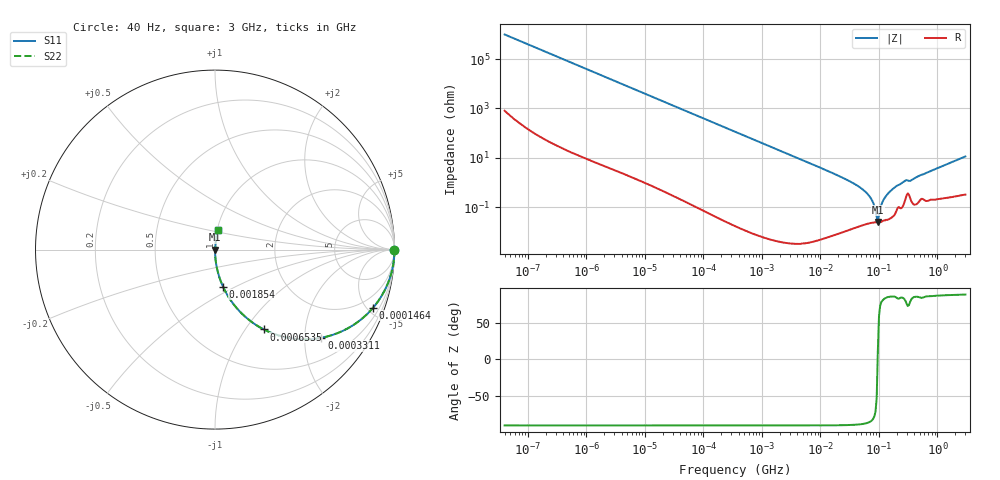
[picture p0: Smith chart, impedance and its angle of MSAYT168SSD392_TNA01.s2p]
! MSAYT168SSD392_TNA01  S-PARAMETER MODEL  ( General Type )
! Model Generated by TAIYO YUDEN Corporation (http://www.ty-top.com)
! Version 2.0
! TAIYO YUDEN Control No. 031107
! Copyright(c) 2003 TAIYO YUDEN CO.,LTD. All Rights Reserved.
! Product Description (link to TY-COMPAS)
! https://ds.yuden.co.jp/TYCOMPAS/or/detail?pn=MSAYT168SSD392KTNA01&u=M
! Products Name : Multilayer Ceramic Capacitors
! Characteristics :
!  Capacitance : 3900 pF , Rated Voltage : 25V
!  Case Size : 1.6 x 0.8 / 0.063 x 0.031 [mm/inch] , Thickness : 0.8 / 0.031 [mm/inch]
!  (Conditions: Temperature = 25 degC , DC Bias Current/Voltage = 0A / 0V)
! External Node Assignments :
!  1  o---| |---o  2
! GND o---------o GND
! Frequency Range : 40Hz  -  3GHz  [ 401 STEP ]
# MHz S RI R 50
! Freq[MHz].  S11 Real  S11 Imag  S21 Real  S21 Imag  S12 Real  S12 Imag  S22 Real  S22 Imag
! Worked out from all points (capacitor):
!   401 points, 40 Hz to 3 GHz, reference 50 ohm
!   read as one part in series: C = 3.98 nF near 44 Hz
!   lowest |Z| = 25.1 mohm at 95.69 MHz (marker M1)
!   series resonance near 95.09 MHz, so ESL is about 700 pH
!   S11 on the Smith chart (normalised r, x): 40 Hz: open; 146.4 kHz: 1.00, -5.46; 331.1 kHz: 1.00, -2.41; 653.5 kHz: 1.00, -1.22; 1.854 MHz: 1.00, -0.43; 3 GHz: 1.01, +0.23
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4e-05  1 -0.0001  9.1e-08 0.0001  9.1e-08 0.0001  1 -0.0001
0.000834  1 -0.00209  4.83e-06 0.00209  4.83e-06 0.00209  1 -0.00209
0.017386  0.9981 -0.0434  0.0019 0.0434  0.0019 0.0434  0.9981 -0.0434
0.056505  0.9804 -0.1386  0.0196 0.1386  0.0196 0.1386  0.9804 -0.1386
0.146395  0.8816 -0.323  0.1184 0.323  0.1184 0.323  0.8816 -0.323
0.331057  0.593 -0.4912  0.407 0.4912  0.407 0.4912  0.593 -0.4912
0.362475  0.5486 -0.4976  0.4514 0.4976  0.4514 0.4976  0.5486 -0.4976
0.653458  0.2722 -0.445  0.7278 0.445  0.7278 0.445  0.2722 -0.445
1.853676  0.0444 -0.2059  0.9556 0.2059  0.9556 0.2059  0.0444 -0.2059
7.222098  0.00306 -0.0548  0.9969 0.0548  0.9969 0.0548  0.00306 -0.0548
26.8909  0.000291 -0.0136  0.9997 0.0136  0.9997 0.0136  0.000291 -0.0136
50.72622  0.000211 -0.00561  0.9998 0.00561  0.9998 0.00561  0.000211 -0.00561
72.90103  0.000234 -0.00225  0.9998 0.00225  0.9998 0.00225  0.000234 -0.00225
79.8195  0.00024 -0.00147  0.9998 0.00147  0.9998 0.00147  0.00024 -0.00147
87.39454  0.000244 -0.000701  0.9998 0.000701  0.9998 0.000701  0.000244 -0.000701
95.68847  0.000246 5.22e-05  0.9998 -5.22e-05  0.9998 -5.22e-05  0.000246 5.22e-05
100.1261  0.000261 0.000434  0.9997 -0.000434  0.9997 -0.000434  0.000261 0.000434
120.0322  0.00029 0.00198  0.9997 -0.00198  0.9997 -0.00198  0.00029 0.00198
150.5692  0.000348 0.00406  0.9997 -0.00406  0.9997 -0.00406  0.000348 0.00406
271.4411  0.00165 0.0111  0.9984 -0.0111  0.9984 -0.0111  0.00165 0.0111
356.2883  0.00192 0.0121  0.9981 -0.0121  0.9981 -0.0121  0.00192 0.0121
3000  0.0159 0.1115  0.9841 -0.1115  0.9841 -0.1115  0.0159 0.1115
